//FC653	Send/Receive Schnittstelle - Empfang
// ***************************************************************************
FUNCTION "FC_SR_RECV" : VOID

TITLE =Send/Receive Empfang

AUTHOR: 	SIEMENS
FAMILY: 	SISTARS7
VERSION: 	4.02

//KNOW_HOW_PROTECT

//Hinweis:
//Der Baustein wird vom FC651 aufgerufen, wenn Daten im Empfangspuffer
//bearbeitet werden sollen. Da im FC651 der Verbindungssatz des DB984
//geladen ist darf er im FC653 nicht veraendert werden

// Datum	 Name			Aktion
// ---------------------------------------------------------------------------
// 19.05.99  Mahler		Neu



//Eingabeparameter
VAR_INPUT
	iFKT			: INT;		//Aufrufmodus
	iVBNR			: INT;		//
END_VAR

//Ausgabeparameter
//VAR_OUTPUT
//END_VAR


//Temporäre/Lokale Variable
VAR_TEMP

	anyQUEL	: ANY; 	         //Offset=0, Zeiger muss an erster Stelle stehen
	anyZIEL	: ANY;		   //Offset=10,
	uVerb		:"XC_INIT_SR_UDT";   //Offset=20
      uJob		:"XC_JOB_SR_UDT";    //Offset=70


      iLoop		: INT;
	iAct		: INT;

	bCSend	: Byte;
	bCRecv	: Byte;
	bCSave	: Byte;

      dwPTR1	: DWORD;
      dwPTR2	: DWORD;

      bZTyp		: Byte;
	bQTyp		: Byte;
	iDB		: INT;
	iDW		: INT;
      iAnz		: INT;

      iRecvDW     : INT;

      iSysJob     : INT;
      iDone		: INT;

      iDW1		: INT;
      iDW2		: INT;
      iDW3		: INT;
      iDW4		: INT;
      iDW5		: INT;
      iDW6		: INT;

	dwAR1			: DWORD;

END_VAR

BEGIN

NETWORK
TITLE = AR1 retten
// ===========================================================================

	TAR1	#dwAR1;


NETWORK
TITLE = Vorbesetzen der Zeiger
// ===========================================================================
//Pionter fuer den Empfangspuffer zusammenstellen
//Any-Pointer:
//Byte 0	: S7-Typ 		= 16=10H                 LB0,LB10
//Byte 1	: Datentyp		= 02=Byte			 LB1,LB11
//Byte 2/3	: Wiederholungsfaktor				 LW2,LW12
//Byte 4/5	: DB-Nummer						 LW4,LW14
//Byte 6-9	: Bereichszeiger					 LD6,LD16

	L 16;		//S7-Typ
	T LB 0;
	T LB 10;
	L 2;		//Datentyp=Byte
	T LB1;
	T LB11;


NETWORK
TITLE =Daten holen	- Verbindungsblock
// ===========================================================================
	L iFKT;
	L 1;
	<>I;
	spb end2;

	L   #iVBNR;
	+  -1;
	L   "XC_VERB_SR".iLen;
      *I;
	L   "XC_VERB_SR".iOffset;
	+I;
	SLD 3;
	T #dwPTR1;		//Bereichszeiger

	LAR1 p#20.0;       //Pionter auf uVERB in den lokalen Daten
	auf  "XC_VERB_SR";

//Schleife um Daten in lokale Variable Byteweise umzuladen
	L  "XC_VERB_SR".iLen;		//Anzahl der Bytes
Lo21: T #iLoop;

      L DBB[#dwPTR1];		//Wert aus DB holen
	T LB [AR1,p#0.0];		//Wert in uVERB eintragen

	+AR1 p#1.0;			//AR1 um 1Bytes erhoehen
	l  #dwPTR1;			//Zeiger fuer DB-Datenwort erhoehen
	L 8;
	+D;
	T #dwPTR1;
	L   #iLoop;			//Schleifenzaehler erniedrigen und zum Anfang
	LOOP Lo21;


end2: nop 0;

NETWORK
TITLE =Zyklischer Teil:  FKT 1 - Datenempfang
// ===========================================================================

	l #iFkt;
	l 1;
	<>I;
      spb end1;

      l #uVerb.iSendDW;
      sld 3; 			//Im Sendepuffer Byte0 steht der alte Tel-Zaehler
      T   #dwPTR1;		//aus dem vorherigen Telegramm

	l #uVerb.iRecvDW;
      sld 3; 			//Im Empfangspuffer Byte1 steht der Tel-Zaehler
      l 8;				//der vom Koppelpartner gesendet wurde
	+d;
	T   #dwPTR2;


	AUF  DB[#uVerb.iRecvDB];
      l   DBB[#dwPTR2];
	t   #bCRecv;                //Telegrammzaehler aus Empfangspuffer  Byte 1

	AUF  DB[#uVerb.iSendDB];
	l   DBB[#dwPTR1];
	t   #bCSend; 		   //Telegrammzaehler aus Sendepuffer  Byte 0


      l   #bCRecv;
	T   DBB[#dwPTR1];		 //Empfangszaehler als Quittung in den Sendepuffer Byte 0

	l   #bCRecv;		//Wenn Zaehler gleich nur Daten ohne Quittung
	l   #bCSend;            //Wenn Zaehler ungleich Daten und Quittung senden ueber Systemjob
	==I;
      spb Data;
//*****************************
//Quittung erforderlich
//*****************************


      L   "XC_JOB_SR".iSys;				//Quittung senden, wenn ein Systemjob moeglich ist
      srw 1;                                    //Es gibt 64 Systemjobs nur 33 ... 64 sind fuer
      + 1;                                      //direkte Systemaufrufe aus dem Programm reserviert
	t #iSysJob;

      l 0;                    //Kennung nicht gefunden
	t #iDone;

Lo30:	L   #iSysJob;			//In einer Schleife nach einem freiem Systemblock suchen
	+  -1;
	L   "XC_JOB_SR".iLen;
      *I;
	L   "XC_JOB_SR".iOffsetSys;
	+I;
	SLD 3;
	T #dwPTR1;		//Bereichszeiger

	LAR1 p#70.0;       //Pionter auf uVERB in den lokalen Daten
	auf  "XC_JOB_SR";

//Schleife um Daten in lokale Variable Byteweise umzuladen
	L  "XC_JOB_SR".iLen;		//Anzahl der Bytes
Lo31: T #iLoop;

      L DBB[#dwPTR1];		//Wert aus DB holen
	T LB [AR1,p#0.0];		//Wert in uVERB eintragen

	+AR1 p#1.0;			//AR1 um 1Bytes erhoehen
	l  #dwPTR1;			//Zeiger fuer DB-Datenwort erhoehen
	L 8;
	+D;
	T #dwPTR1;
	L   #iLoop;			//Schleifenzaehler erniedrigen und zum Anfang
	LOOP Lo31;

	u #uJob.boEnable;        //Pruefen ob Block belegt
	spb  ne31;
      s #uJob.boEnable;
      s #uJob.boTmpJob;

	L 1;				//Kennung eingetragen
	t #iDone;

	u #uVerb.boS5;		//Pruefen ob Partner eine S5-Steuerung
	spb s5;

	l  985;			//Ziel-DB = 985 bei S7
	t  #uJob.iDest_DB;
      spb quda;

s5:	l  205;			//Ziel-DB = 985 bei S7
	t  #uJob.iDest_DB;


quda: L #uVerb.bPCU;          //PCU-Nummer eintragen
      t #uJob.iPCU;

      L 50;                   //Auftragstyp = DB senden
	t #uJob.bType;

      L 2;                    //Datentyp = 2Bytes
	t  #uJob.bSrc_DType;
	t  #uJob.bDest_DType;

	L B#16#84;              //Bereich = 84=DB
	t  #uJob.bSrc_AREA;
	t  #uJob.bDest_AREA;

	L  985;              	//Quell-DB = 985
	t  #uJob.iSrc_DB;

	l 0;				//DW = 0
	t #uJob.dwSrcByte;
	t #uJob.dwDestByte;

	l 2;				//Anzahl Bytes
	t #uJob.iSrc_Num;
	t #uJob.iDest_Num;


ne31:	L   #iSysJob;			//In einer Schleife Systemblock zurueckschreiben
	+  -1;
	L   "XC_JOB_SR".iLen;
      *I;
	L   "XC_JOB_SR".iOffsetSys;
	+I;
	SLD 3;
	T #dwPTR1;		//Bereichszeiger

	LAR1 p#70.0;       //Pionter auf uJob in den lokalen Daten

	L  "XC_JOB_SR".iLen;		//Anzahl der Bytes
Lo32: T #iLoop;

  	l LB [AR1,p#0.0];		//Wert in uJob eintragen
      T DBB[#dwPTR1];		//Wert aus DB holen

	+AR1 p#1.0;			//AR1 um 1Bytes erhoehen
	l  #dwPTR1;			//Zeiger fuer DB-Datenwort erhoehen
	L 8;
	+D;
	T #dwPTR1;
	L   #iLoop;			//Schleifenzaehler erniedrigen und zum Anfang
	LOOP Lo32;

	l #iDone;			//Pruefen ob Eintrag erfolgt ist
      l 1;
	==I;
	spb Data;

      l   #iSysJob;			//Naechsten Systemjob anwaehlen
      inc 1;
      t   #iSysJob;
	L   "XC_JOB_SR".iSys;
      <=I;
      spb Lo30;


//*******************************
//Empfangspuffer entsorgen
//*******************************

Data: Nop 0;                 //Empfangspuffer entsorgen

	L 2;
	t #iAct;                  //Zeiger auf Anfang Header

DA11: l #uVerb.iRecvDW;
      l #iAct;
	+I;
	sld 3;
      T   #dwPTR1;

      auf DB[#uVerb.iRecvDB];
	L  DBW[#dwPTR1];		//Bei Endekennung dh. -1 fertig
      l  -1;
	==I;
 	spb end1;

	l #uVerb.iRecvDW;       //Zeiger Anfang Empfangspuffer
      l #iAct;	            // + Offset auf Block
	+I;				// + 8 Bytes Header
	L 8;
	+I;
      t #iRecvDW;             //Anfang Nutzdaten

	l DBB[#dwPTR1];		//Header aus Empfangspuffer   Typ
	t #bZTyp;

	l #dwPTR1;
	l 8;
	+d;
	t #dwPTR1;

	l DBB[#dwPTR1];		//Header aus Empfangspuffer   Typ
	t #bQTyp;

	l #dwPTR1;
	l 8;
	+d;
	t #dwPTR1;

      l  DBW[#dwPTR1];		//Header aus Empfangspuffer  DB
	t #iDB;

	l #dwPTR1;
	l 16;
	+d;
	t #dwPTR1;

      l  DBW[#dwPTR1];		//Header aus Empfangspuffer  DW
	t #iDW;

	l #dwPTR1;
	l 16;
	+d;
	t #dwPTR1;

      l  DBW[#dwPTR1];		//Header aus Empfangspuffer  Anzahl
	slw 1;
      t #iAnz;			//Anzahl in Bytes

	l #bZTyp;			//DB empfangen
      l 50;
      ==I;
      spb copy;

	l #bZTyp;			//DX empfangen da S7 ist Datenziel trotzdem DB
      l 51;
      ==I;
      spb copy;

	l #bZTyp;			//Uhr empfangen
      l 68;
      ==I;
      spb uhr;

	l #bQTyp;			//DB fetch
      l 52;
      ==I;
      spb fetc;
	l #bQTyp;			//DX fetch
      l 53;
      ==I;
      spb fetc;

	l #bZTyp;			//Kettenstart
      l 54;
      ==I;
      spb Kett;
      spa next;               //Typ nicht bekannt

uhr:  l #dwPTR1;
	l 16;
	+d;
	t #dwPTR1;

      L  DBW[#dwPTR1];        //Hsec muessen ungleich Null sein
      l  W#16#0001;
      ow;
      T  DBW[#dwPTR1];

	l #dwPTR1;
	l 16;
	+d;
	t #dwPTR1;
	L  DBW[#dwPTR1];        //24-Stundenformat erzwingen
      l  W#16#bFFF;		//dh. Bit 15=1 Bit 14=0
      uw;
      l  W#16#8000;
      ow;
      T  DBW[#dwPTR1];


copy:  call "FC_COPY" (
                      iQDB	:=#uVerb.iRecvDB,
			    iQDW	:=#iRecvDW,
                      bQTyp   :=b#16#84,
			    iZDB	:=#iDB,
		          iZDW	:=#iDW,
			    bZTyp   :=b#16#84,
			    iLenByte:=#iAnz
			    );

      l #iAnz;   //Fehler beim Kopieren
      l 0;
	==I;
      spb end1;
      spa next;

fetc: nop 0;

    	l #dwPTR1;
	l 16;
	+d;
	t #dwPTR1;
	L  DBW[#dwPTR1];
      T #iDW1;			//ZTyp, QTyp

	l #dwPTR1;
	l 16;
	+d;
	t #dwPTR1;
	L  DBW[#dwPTR1];
      T #iDW2;			//ZDB

	l #dwPTR1;
	l 16;
	+d;
	t #dwPTR1;
	L  DBW[#dwPTR1];
      T #iDW3;			//ZDW

	l #dwPTR1;
	l 16;
	+d;
	t #dwPTR1;
	L  DBW[#dwPTR1];
      T #iDW4;			//Anzahl

	l #dwPTR1;
	l 16;
	+d;
	t #dwPTR1;
	L  DBW[#dwPTR1];
      T #iDW5;			//QDB

	l #dwPTR1;
	l 16;
	+d;
	t #dwPTR1;
	L  DBW[#dwPTR1];
      T #iDW6;			//QDW


 	L   "XC_JOB_SR".iSys;	//Fetch senden, wenn ein Systemjob moeglich ist
      srw 1;			//Bei 64 Jobs ist 33 - 64 fuer das System reserviert
	+ 1;				//dh. immer die obere Hälfte aller Systemjobs
	t #iSysJob;

      l 0;                    //Kennung nicht gefunden
	t #iDone;

Lo34:	L   #iSysJob;			//In einer Schleife nach einem freiem Systemblock suchen
	+  -1;
	L   "XC_JOB_SR".iLen;
      *I;
	L   "XC_JOB_SR".iOffsetSys;
	+I;
	SLD 3;
	T #dwPTR1;		//Bereichszeiger

	LAR1 p#70.0;       //Pionter auf uVERB in den lokalen Daten
	auf  "XC_JOB_SR";

//Schleife um Daten in lokale Variable Byteweise umzuladen
	L  "XC_JOB_SR".iLen;		//Anzahl der Bytes
Lo35: T #iLoop;

      L DBB[#dwPTR1];		//Wert aus DB holen
	T LB [AR1,p#0.0];		//Wert in uVERB eintragen

	+AR1 p#1.0;			//AR1 um 1Bytes erhoehen
	l  #dwPTR1;			//Zeiger fuer DB-Datenwort erhoehen
	L 8;
	+D;
	T #dwPTR1;
	L   #iLoop;			//Schleifenzaehler erniedrigen und zum Anfang
	LOOP Lo35;

	u #uJob.boEnable;        //Pruefen ob Block belegt
	spb  ne32;
      s #uJob.boEnable;
      s #uJob.boTmpJob;

	L 1;				//Kennung eingetragen
	t #iAnz;


      L #uVerb.bPCU;          //PCU-Nummer eintragen
      t #uJob.iPCU;

      L #iDW1;                   //Auftragstyp = DB senden
	srw 8;     			   //Aus Fetch 52/53 wird Sende DB=50 oder DX=51
	+ -2;
      t #uJob.bType;

      L 2;                    //Datentyp = 2Bytes
	t  #uJob.bSrc_DType;
	t  #uJob.bDest_DType;

	L B#16#84;              //Bereich = 84=DB
	t  #uJob.bSrc_AREA;
	t  #uJob.bDest_AREA;

	l  #iDW2;			//Ziel-DB
	t  #uJob.iDest_DB;
	L  #iDW5;              	//Quell-DB
	t  #uJob.iSrc_DB;

	l  #iDW6;			//Quell-DW
	t #uJob.dwSrcByte;
      l #iDW3;			//Ziel-DW
	t #uJob.dwDestByte;

	l  #iDW4;			//Anzahl Bytes
	slw 1;
	t #uJob.iSrc_Num;
	t #uJob.iDest_Num;

      l 1;				//Kennung Auftrag bearbeitet
      t #iDone;

ne32:	L   #iSysJob;			//In einer Schleife Systemblock zurueckschreiben
	+  -1;
	L   "XC_JOB_SR".iLen;
      *I;
	L   "XC_JOB_SR".iOffsetSys;
	+I;
	SLD 3;
	T #dwPTR1;		//Bereichszeiger

	LAR1 p#70.0;       //Pionter auf uJob in den lokalen Daten

	L  "XC_JOB_SR".iLen;		//Anzahl der Bytes
Lo33: T #iLoop;

  	l LB [AR1,p#0.0];		//Wert in uJob eintragen
      T DBB[#dwPTR1];		//Wert aus DB holen

	+AR1 p#1.0;			//AR1 um 1Bytes erhoehen
	l  #dwPTR1;			//Zeiger fuer DB-Datenwort erhoehen
	L 8;
	+D;
	T #dwPTR1;
	L   #iLoop;			//Schleifenzaehler erniedrigen und zum Anfang
	LOOP Lo33;

	l #iDone;			//Pruefen ob Eintrag erfolgt ist
      l 1;
	==I;
	spb next;

      l   #iSysJob;			//Naechsten Systemjob anwaehlen
      inc 1;
      t   #iSysJob;
	L   "XC_JOB_SR".iSys;
      <=I;
      spb Lo34;

      spa next;


Kett:  nop 0;

	Auf DB[#uVerb.iRecvDB];
	l  #dwPTR1;
	l 16;
	+d;
	t #dwPTR1;
	L  DBW[#dwPTR1];
      T #iDW1;			//Starttyp

	l #dwPTR1;
	l 16;
	+d;
	t #dwPTR1;
	L  DBW[#dwPTR1];
      T #iDW2;			//Quellteilanlage

	l #dwPTR1;
	l 16;
	+d;
	t #dwPTR1;
	L  DBW[#dwPTR1];
      T #iDW3;			//Rezepttyp

	l #dwPTR1;
	l 16;
	+d;
	t #dwPTR1;
	L  DBW[#dwPTR1];
      T #iDW4;			//Rezeptnummer

	l #dwPTR1;
	l 16;
	+d;
	t #dwPTR1;
	L  DBW[#dwPTR1];
      T #iDW5;			//Auftragsnummer

	l #dwPTR1;
	l 16;
	+d;
	t #dwPTR1;
	L  DBW[#dwPTR1];
      T #iDW6;			//Chargennummer

	Auf "XC_RASTA_SR";
	l #bQTyp;			//Ziel-Teilanlage
      + -1;
	L "XC_RASTA_SR".iLen;
      *I;
	l "XC_RASTA_SR".iOffset;
      +I;
	SLd 3;
	LAR1;

	L uVerb.bPCU;		//Quell-PCU in ASTA
	T   DBB[AR1,p#0.0];
      T   DBB[AR1,p#1.0];

	L #iDW2;			//Quell-ASTA in ASTA
	T   DBB[AR1,p#2.0];

	l #bQTyp;
	T   DBB[AR1,p#3.0];	//Ziel-Teilanlage in ASTA

	l #iDW3;
	T   DbW[AR1,p#4.0];	//Jahr,Rezepttyp in ASTA
	l #iDW4;
	T   DbW[AR1,p#6.0];	//Rezeptnummer in ASTA
	l #iDW5;
	T   Dbw[AR1,p#8.0];	//Auftragsnummer in ASTA
	l #iDW6;
	T   Dbw[AR1,p#10.0];	//Chargennummer in ASTA

	U  uverb.boS5;
	spb s5K;
	u  uverb.boS7;
	spb s7K;
	spb next;
s5K:	call fc 654 (			//Teilanlage starten Tel. von S5
			iFkt	:=52
			);
	spa  next;
s7K:	call fc 654 (			//Teilanlage starten Tel. von S7
			iFkt	:=72
			);

      spa next;

next: l #iAnz;			//Anzahl Nutzdaten in Bytes
      + 8; 			     //Anzahl 8 Bytes Header
	l #iAct;
      +I;
	t #iAct;


      l #iAct;			//Pruefen ob noch Platz im Empfangspuffer
      l 10;                   //Auftrag mindestens 5 DW  dh. 4*Header + 1*Endekennung
      +I;
	l #uVerb.iLen;
      <=I;
	spb DA11;


end1: nop 0;

NETWORK
TITLE = AR1 zurück, ENDE
// ===========================================================================

	LAR1	#dwAR1;

END_FUNCTION
